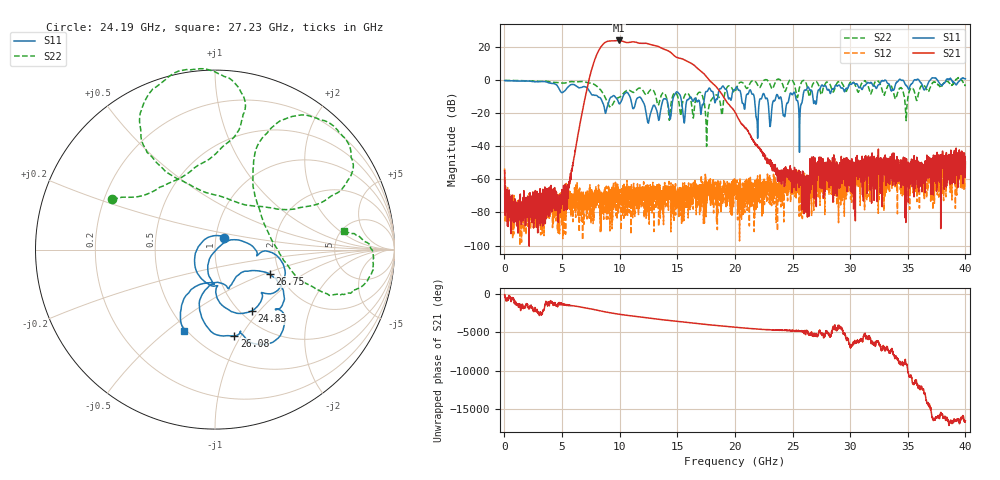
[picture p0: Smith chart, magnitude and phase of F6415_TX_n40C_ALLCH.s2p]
!Keysight Technologies,N5245B,MY52451815,A.15.70.20
!Date: Thursday, April 18, 2024 10:50:33
!Correction: S33(C  2-Port  )
!S43(C  2-Port  )
!S34(C  2-Port  )
!S44(C  2-Port  )
!S2P File: Measurements: S33, S43, S34, S44:
# Hz S  RI  R 50
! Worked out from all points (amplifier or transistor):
!   4000 points, 10 MHz to 40 GHz, reference 50 ohm
!   highest |S21| = 23.7 dB at 9.9 GHz (marker M1)
!   |S21| within 3 dB of that: 8.46 GHz to 13.01 GHz (4.547 GHz wide, 42.4 % of centre)
!   unconditionally stable (mu >= 1): start of sweep to 22.61 GHz; 24.92 GHz to 34.24 GHz; 34.39 GHz to 35.6 GHz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
!   at 6.67 GHz: K = 3799.90, MAG = -13.8 dB, |S12| = -72.3 dB
!   at 20.01 GHz: K = 8929.06, MAG = -17.4 dB, |S12| = -69.9 dB
!   at 40 GHz: K = -5642.03, MSG = 2.4 dB, |S12| = -54.4 dB
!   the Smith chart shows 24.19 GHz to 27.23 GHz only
!   S11 on the Smith chart (normalised r, x): 24.19 GHz: 1.10, +0.15; 24.83 GHz: 1.12, -0.91; 26.08 GHz: 0.74, -0.94; 26.75 GHz: 1.77, -0.54; 27.23 GHz: 0.49, -0.58
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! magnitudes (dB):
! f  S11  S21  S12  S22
! 10 MHz  -0.5  -54.9  -53.5  -0.4
! 550 MHz  -0.7  -86.1  -86.9  -0.5
! 4.7 GHz  -5.0  -75.1  -72.2  -1.7
! 5.51 GHz  -4.4  -63.6  -76.1  -1.5
! 6.68 GHz  -4.7  -21.9  -85.2  -1.1
! 8.12 GHz  -10.3  16.9  -66.1  -4.6
! 9.9 GHz  -13.7  23.7  -66.2  -10.8
! 13.34 GHz  -23.1  20.1  -77.4  -15.3
! 14.96 GHz  -7.3  13.4  -69.0  -8.9
! 16.96 GHz  -15.1  5.6  -66.4  -7.6
! 17.57 GHz  -7.1  1.5  -74.2  -31.6
! 20.01 GHz  -5.8  -19.6  -69.9  -7.4
! 24.19 GHz  -21.5  -60.6  -61.0  -3.9
! 24.83 GHz  -8.0  -55.1  -73.9  0.1
! 25.66 GHz  -18.9  -55.5  -66.4  -3.2
! 26.08 GHz  -6.1  -66.9  -61.4  -0.8
! 26.67 GHz  -6.6  -51.3  -55.4  -4.3
! 26.75 GHz  -9.6  -48.2  -71.6  -2.7
! 27.23 GHz  -6.3  -49.6  -59.5  -2.8
! 33.34 GHz  -2.4  -61.7  -65.6  -3.1
! 34.85 GHz  -3.5  -65.7  -56.0  -24.4
! 40 GHz  0.5  -49.6  -54.4  -3.4
